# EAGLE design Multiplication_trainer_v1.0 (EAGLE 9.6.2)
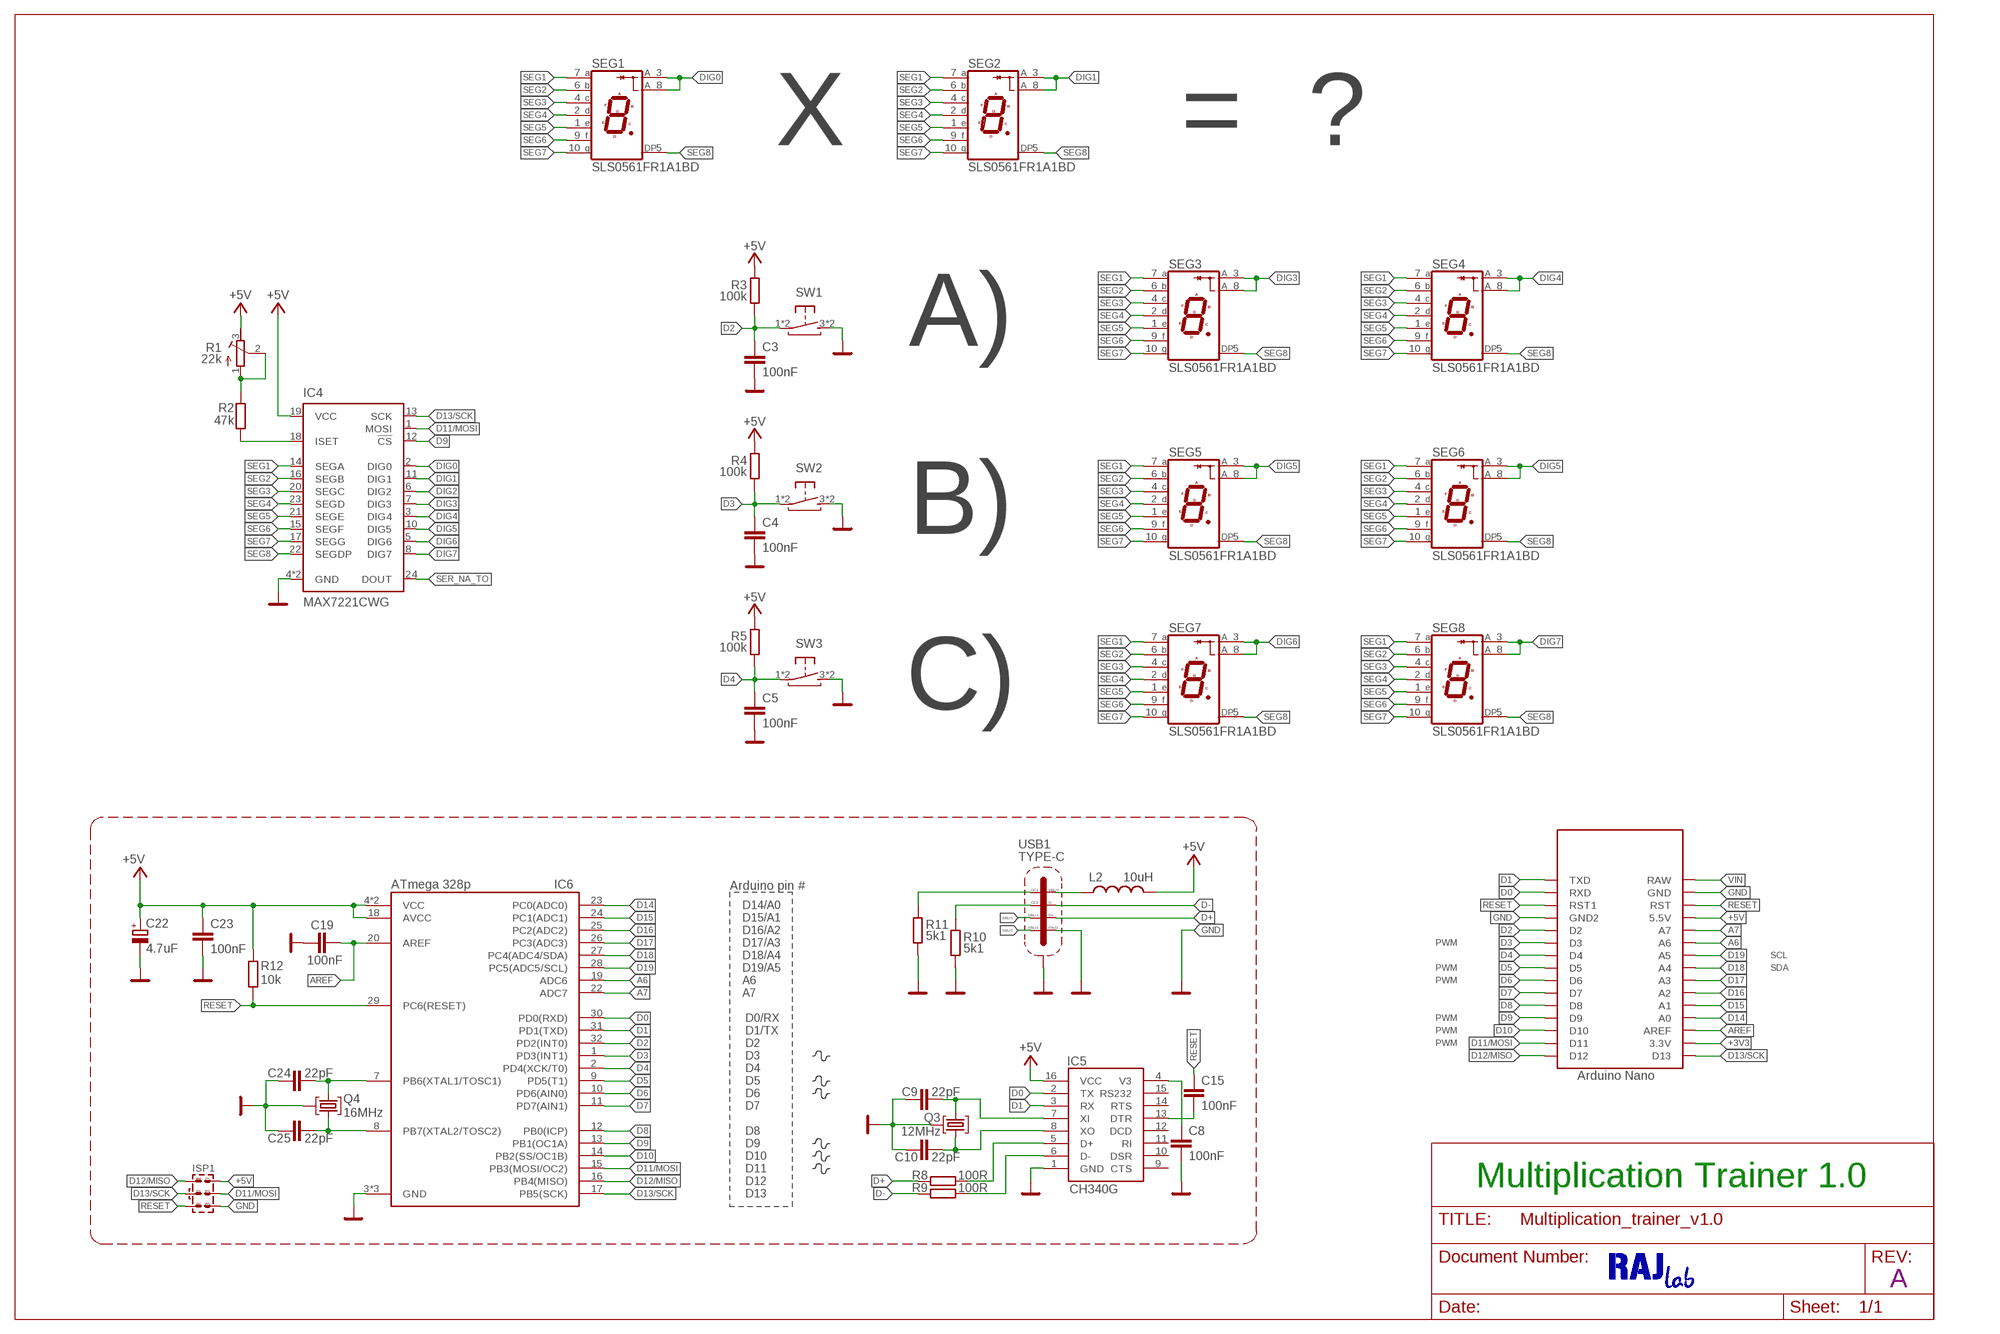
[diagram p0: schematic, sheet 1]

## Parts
C3  100nF  C-EUC0805  [C0805]
C4  100nF  C-EUC0805  [C0805]
C5  100nF  C-EUC0805  [C0805]
C8  100nF  C-EUC0603  [C0603]
C9  22pF  C-EUC0603  [C0603]
C10  22pF  C-EUC0603  [C0603]
C15  100nF  C-EUC0603  [C0603]
C19  100nF  C-EUC0603  [C0603]
C22  4.7uF  CPOL-EUSMCA  [SMC_A]
C23  100nF  C-EUC0603  [C0603]
C24  22pF  C-EUC0603  [C0603]
C25  22pF  C-EUC0603  [C0603]
IC4  MAX7221CWG  [SOIC127P1032X265-24N]
IC5  CH340G  CH340GSMD  [SOIC16]
IC6  ATmega 328p  ATMEGA328PQFP32N_ROUND-PADS  [QFP80P900X900X120-32N_ROUND-PADS]
ISP1  AVR-ISP-SPI  [AVR-ISP-SPI]
L2  10uH  L-USL0805  [R0805]
Q3  12MHz  KRYSTAL  [ILCX13-FF5F18-16.0000]
Q4  16MHz  KRYSTAL  [ILCX13-FF5F18-16.0000]
R1  22k  R-TRIMM3305  [RTRIM3305]
R2  47k  R-EU_R0805  [R0805]
R3  100k  R-EU_R0805  [R0805]
R4  100k  R-EU_R0805  [R0805]
R5  100k  R-EU_R0805  [R0805]
R8  100R  R-EU_R0603  [R0603]
R9  100R  R-EU_R0603  [R0603]
R10  5k1  R-EU_R0603  [R0603]
R11  5k1  R-EU_R0603  [R0603]
R12  10k  R-EU_R0603  [R0603]
SEG1  SLS0561FR1A1BD  [SLS0561FR1A1BD]
SEG2  SLS0561FR1A1BD  [SLS0561FR1A1BD]
SEG3  SLS0561FR1A1BD  [SLS0561FR1A1BD]
SEG4  SLS0561FR1A1BD  [SLS0561FR1A1BD]
SEG5  SLS0561FR1A1BD  [SLS0561FR1A1BD]
SEG6  SLS0561FR1A1BD  [SLS0561FR1A1BD]
SEG7  SLS0561FR1A1BD  [SLS0561FR1A1BD]
SEG8  SLS0561FR1A1BD  [SLS0561FR1A1BD]
SW1  TACT-SW_BTNSMTJLC_6X6X4.5  [TACTSW_6X6X4.5_SMT]
SW2  TACT-SW_BTNSMTJLC_6X6X4.5  [TACTSW_6X6X4.5_SMT]
SW3  TACT-SW_BTNSMTJLC_6X6X4.5  [TACTSW_6X6X4.5_SMT]
U$2  NANOTHT-NOUSB  [NANO-NOUSB]
USB1  TYPE-C  TYPE-C-31-M-12TYPE-C-31_L8.94_W7.3  [TYPE-C-31_L8.94_W7.3]

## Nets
+3V3: U$2.3.3V
+5V: C22.+ C23.1 IC4.19(VCC) IC5.16(VCC) IC6.4(VCC) IC6.6(VCC) IC6.18(AVCC) ISP1.2 L2.2 R1.3(E) R3.1 R4.1 R5.1 R12.1 U$2.5V(5.5V)
A6: IC6.19(ADC6) U$2.A6
A7: IC6.22(ADC7) U$2.A7
AREF: C19.1 IC6.20(AREF) U$2.AREF
D0: IC5.2(TX) IC6.30(PD0(RXD)) U$2.RX1(RXD)
D1: IC5.3(RX) IC6.31(PD1(TXD)) U$2.TX0(TXD)
D2: C3.1 IC6.32(PD2(INT0)) R3.2 SW1.1(P) SW1.2(P) U$2.D2
D3: C4.1 IC6.1(PD3(INT1)) R4.2 SW2.1(P) SW2.2(P) U$2.D3
D4: C5.1 IC6.2(PD4(XCK/T0)) R5.2 SW3.1(P) SW3.2(P) U$2.D4
D5: IC6.9(PD5(T1)) U$2.D5
D6: IC6.10(PD6(AIN0)) U$2.D6
D7: IC6.11(PD7(AIN1)) U$2.D7
D8: IC6.12(PB0(ICP)) U$2.D8
D9: IC4.12(!CS) IC6.13(PB1(OC1A)) U$2.D9
D10: IC6.14(PB2(SS/OC1B)) U$2.D10
D11/MOSI: IC4.1(MOSI) IC6.15(PB3(MOSI/OC2)) ISP1.4 U$2.D11
D12/MISO: IC6.16(PB4(MISO)) ISP1.1 U$2.D12
D13/SCK: IC4.13(SCK) IC6.17(PB5(SCK)) ISP1.3 U$2.D13
D14: IC6.23(PC0(ADC0)) U$2.A0
D15: IC6.24(PC1(ADC1)) U$2.A1
D16: IC6.25(PC2(ADC2)) U$2.A2
D17: IC6.26(PC3(ADC3)) U$2.A3
D18: IC6.27(PC4(ADC4/SDA)) U$2.A4
D19: IC6.28(PC5(ADC5/SCL)) U$2.A5
D+: R8.1 USB1.A6(D+) USB1.B6(D+)
D-: R9.1 USB1.A7(D-) USB1.B7(D-)
DIG0: IC4.2(DIG0) SEG1.3(CA1) SEG1.8(CA2)
DIG1: IC4.11(DIG1) SEG2.3(CA1) SEG2.8(CA2)
DIG2: IC4.6(DIG2)
DIG3: IC4.7(DIG3) SEG3.3(CA1) SEG3.8(CA2)
DIG4: IC4.3(DIG4) SEG4.3(CA1) SEG4.8(CA2)
DIG5: IC4.10(DIG5) SEG5.3(CA1) SEG5.8(CA2) SEG6.3(CA1) SEG6.8(CA2)
DIG6: IC4.5(DIG6) SEG7.3(CA1) SEG7.8(CA2)
DIG7: IC4.8(DIG7) SEG8.3(CA1) SEG8.8(CA2)
GND: C3.2 C4.2 C5.2 C8.2 C9.2 C10.2 C19.2 C22.- C23.2 C24.2 C25.2 IC4.4(GND) IC4.9(GND) IC5.1(GND) IC6.3(GND) IC6.5(GND) IC6.21(GND) ISP1.6 Q3.P$2(GND) Q3.P$4(GND) Q4.P$2(GND) Q4.P$4(GND) R10.1 R11.1 SW1.3(S) SW1.4(S) SW2.3(S) SW2.4(S) SW3.3(S) SW3.4(S) U$2.GND U$2.GND1(GND2) USB1.A1/B12(GND) USB1.B1/A12(GND) USB1.SHIELD1(SHIELD) USB1.SHIELD2(SHIELD) USB1.SHIELD3(SHIELD) USB1.SHIELD4(SHIELD) USB1.SHIELD5(SHIELD) USB1.SHIELD6(SHIELD) USB1.SHIELD7(SHIELD) USB1.SHIELD8(SHIELD)
N$1: C8.1 IC5.4(V3)
N$2: C9.1 IC5.7(XI) Q3.P$1
N$3: C10.1 IC5.8(XO) Q3.P$3
N$4: C15.2 IC5.13(DTR)
N$5: IC5.5(D+) R8.2
N$6: IC4.18(ISET) R2.1
N$7: R1.1(A) R1.2(S) R2.2
N$8: IC5.6(D-) R9.2
N$9: L2.1 USB1.A4/B9(VBUS) USB1.B4/A9(VBUS)
N$10: R10.2 USB1.B5(CC2)
N$11: R11.2 USB1.A5(CC1)
N$12: C24.1 IC6.7(PB6(XTAL1/TOSC1)) Q4.P$1
N$13: C25.1 IC6.8(PB7(XTAL2/TOSC2)) Q4.P$3
RESET: C15.1 IC6.29(PC6(RESET)) ISP1.5 R12.2 U$2.RST U$2.RST1
SBU1: USB1.A8(SBU1)
SBU2: USB1.B8(SBU2)
SEG1: IC4.14(SEGA) SEG1.7(A) SEG2.7(A) SEG3.7(A) SEG4.7(A) SEG5.7(A) SEG6.7(A) SEG7.7(A) SEG8.7(A)
SEG2: IC4.16(SEGB) SEG1.6(B) SEG2.6(B) SEG3.6(B) SEG4.6(B) SEG5.6(B) SEG6.6(B) SEG7.6(B) SEG8.6(B)
SEG3: IC4.20(SEGC) SEG1.4(C) SEG2.4(C) SEG3.4(C) SEG4.4(C) SEG5.4(C) SEG6.4(C) SEG7.4(C) SEG8.4(C)
SEG4: IC4.23(SEGD) SEG1.2(D) SEG2.2(D) SEG3.2(D) SEG4.2(D) SEG5.2(D) SEG6.2(D) SEG7.2(D) SEG8.2(D)
SEG5: IC4.21(SEGE) SEG1.1(E) SEG2.1(E) SEG3.1(E) SEG4.1(E) SEG5.1(E) SEG6.1(E) SEG7.1(E) SEG8.1(E)
SEG6: IC4.15(SEGF) SEG1.9(F) SEG2.9(F) SEG3.9(F) SEG4.9(F) SEG5.9(F) SEG6.9(F) SEG7.9(F) SEG8.9(F)
SEG7: IC4.17(SEGG) SEG1.10(G) SEG2.10(G) SEG3.10(G) SEG4.10(G) SEG5.10(G) SEG6.10(G) SEG7.10(G) SEG8.10(G)
SEG8: IC4.22(SEGDP) SEG1.5(DP) SEG2.5(DP) SEG3.5(DP) SEG4.5(DP) SEG5.5(DP) SEG6.5(DP) SEG7.5(DP) SEG8.5(DP)
SER_NA_TO: IC4.24(DOUT)
VIN: U$2.RAW
Unconnected: IC5.9(CTS) IC5.10(DSR) IC5.11(RI) IC5.12(DCD) IC5.14(RTS) IC5.15(RS232)

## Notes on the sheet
- X | = | ?
- A)
- B)
- C)
- Arduino pin #
- D14/A0
- D15/A1
- D16/A2
- D17/A3 | PWM
- D18/A4 | SCL
- D19/A5 | PWM | SDA
- A6 | PWM
- A7
- D0/RX | PWM
- D1/TX | PWM
- D2 | PWM
- D3
- D4
- D5
- D6
- D7
- D8
- D9
- D10
- D11
- D12
- Multiplication Trainer 1.0
- D13
- A

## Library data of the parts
C3-C5 = rcl:C-EU: CAPACITOR, European symbol
C8 C15 C19 C23 = rcl:C-EU: CAPACITOR, European symbol; LCSC_PART: C49678; SPICEPREFIX: C
C9 C10 C24 C25 = rcl:C-EU: CAPACITOR, European symbol; LCSC_PART: C1804; SPICEPREFIX: C
C22 = rcl:CPOL-EU: POLARIZED CAPACITOR, European symbol; LCSC_PART: C111040; ROT: 180; SPICEPREFIX: C
IC4 = MAX7221:MAX7221CWG: 7 SEGMENT 8 DIGIT DRIVER 24SOIC Datasheet; MOUSER_NO: 710-157119S12701
IC5 = ch340g:CH340G; LCSC_PART: C14267
IC6 = ATMEGA328P-ANR:ATMEGA328P: 8-bit Microcontrollers - MCU AVR 32K FLSH 2K SRAM 1KB EE-20 MHZ 105C Source: Datasheet; LCSC_PART: C14877; ROT: 270
ISP1 = #Ondra2:AVR-ISP-SPI
L2 = rcl:L-US: INDUCTOR, American symbol; LCSC_PART: C281113
Q3 = #Marek:KRYSTAL: Monolithic Crystal Filters Source: www.vanlong.com; LCSC_PART: C9002
Q4 = #Marek:KRYSTAL: Monolithic Crystal Filters Source: www.vanlong.com; LCSC_PART: C13738
R1 = rcl:R-TRIMM: Trimm resistor
R2 R8 R9 R12 = rcl:R-EU_: RESISTOR, European symbol; SPICEPREFIX: R
R3-R5 = resistor:R-EU_: RESISTOR, European symbol
R10 R11 = rcl:R-EU_: RESISTOR, European symbol; LCSC_PART: C27834; SPICEPREFIX: R
SEG1-SEG8 = #my:SLS0561FR1A1BD; LCSC_PART: C226002
SW1-SW3 = #Ondra2:TACT-SW_BTN; LCSC_PART: C127509
U$2 = Arduino-clone:NANO: Arduino Nano
USB1 = #Marek:TYPE-C-31-M-12; LCSC_PART: C165948; ROT: 180

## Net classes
0 default: width 0.127 mm, drill 0.2 mm, clearance 0.127 mm

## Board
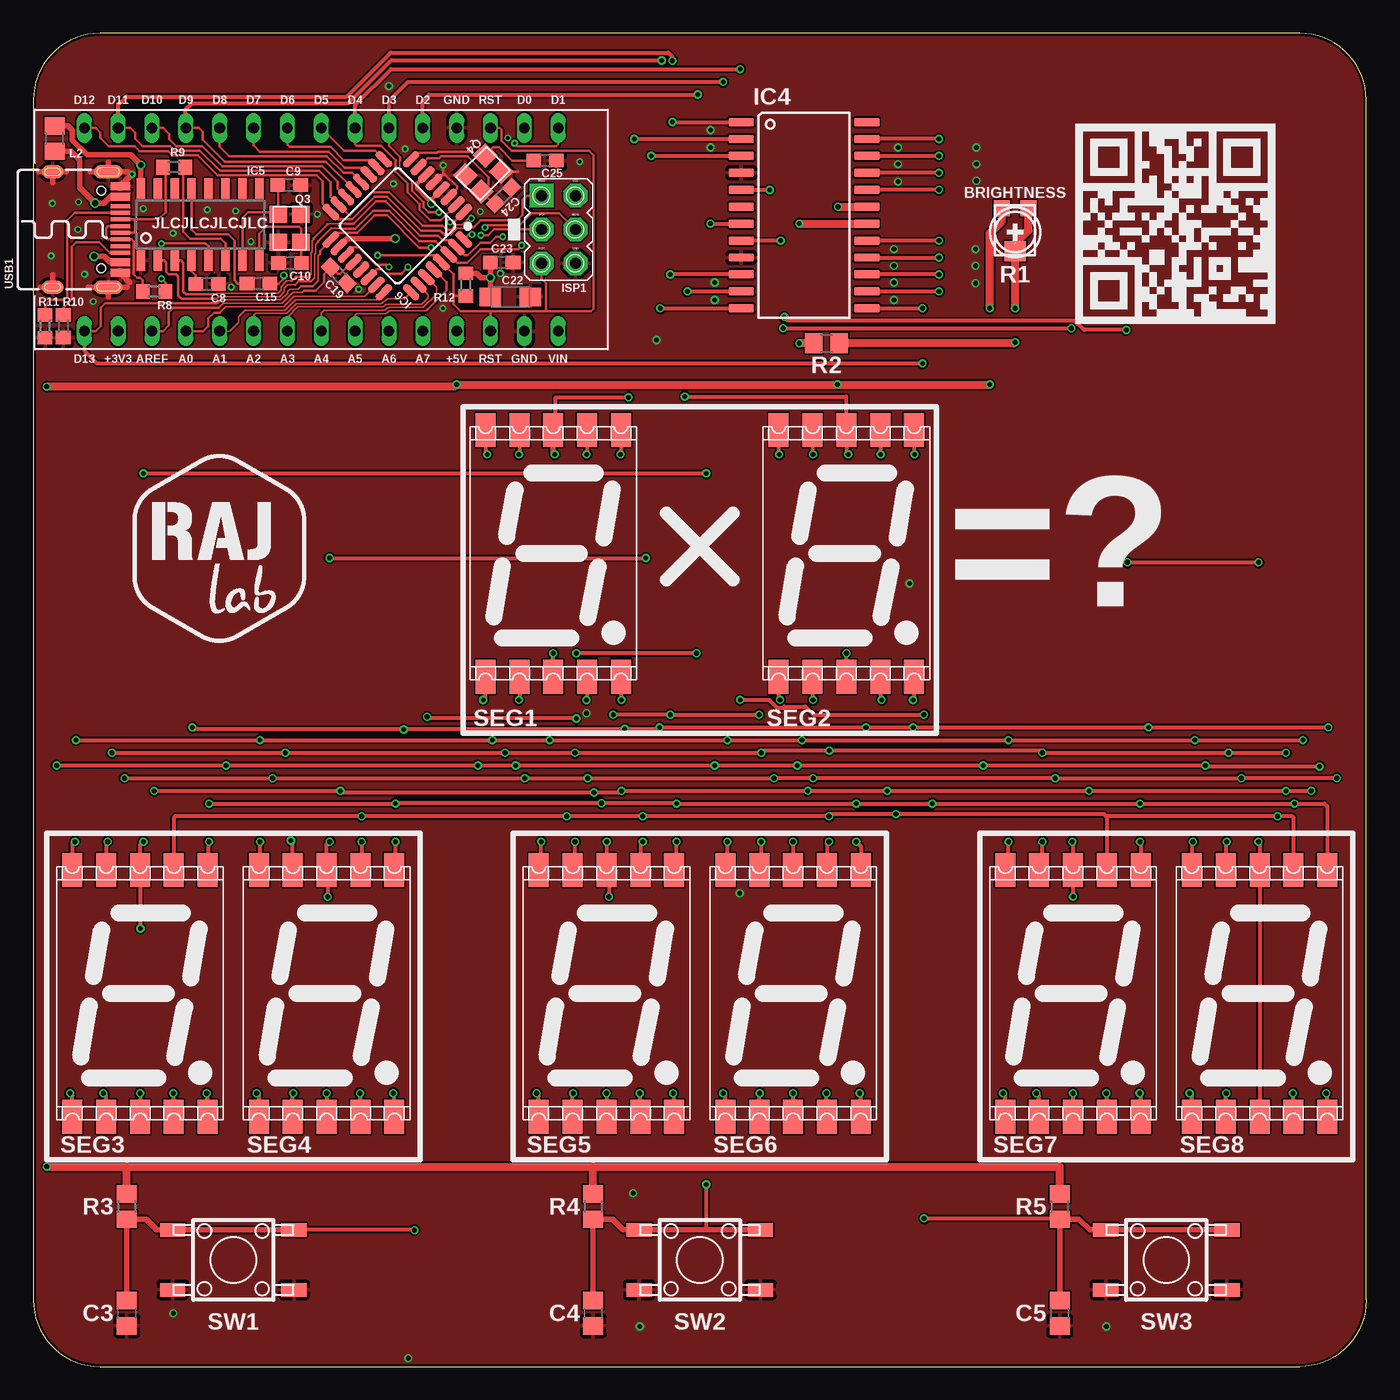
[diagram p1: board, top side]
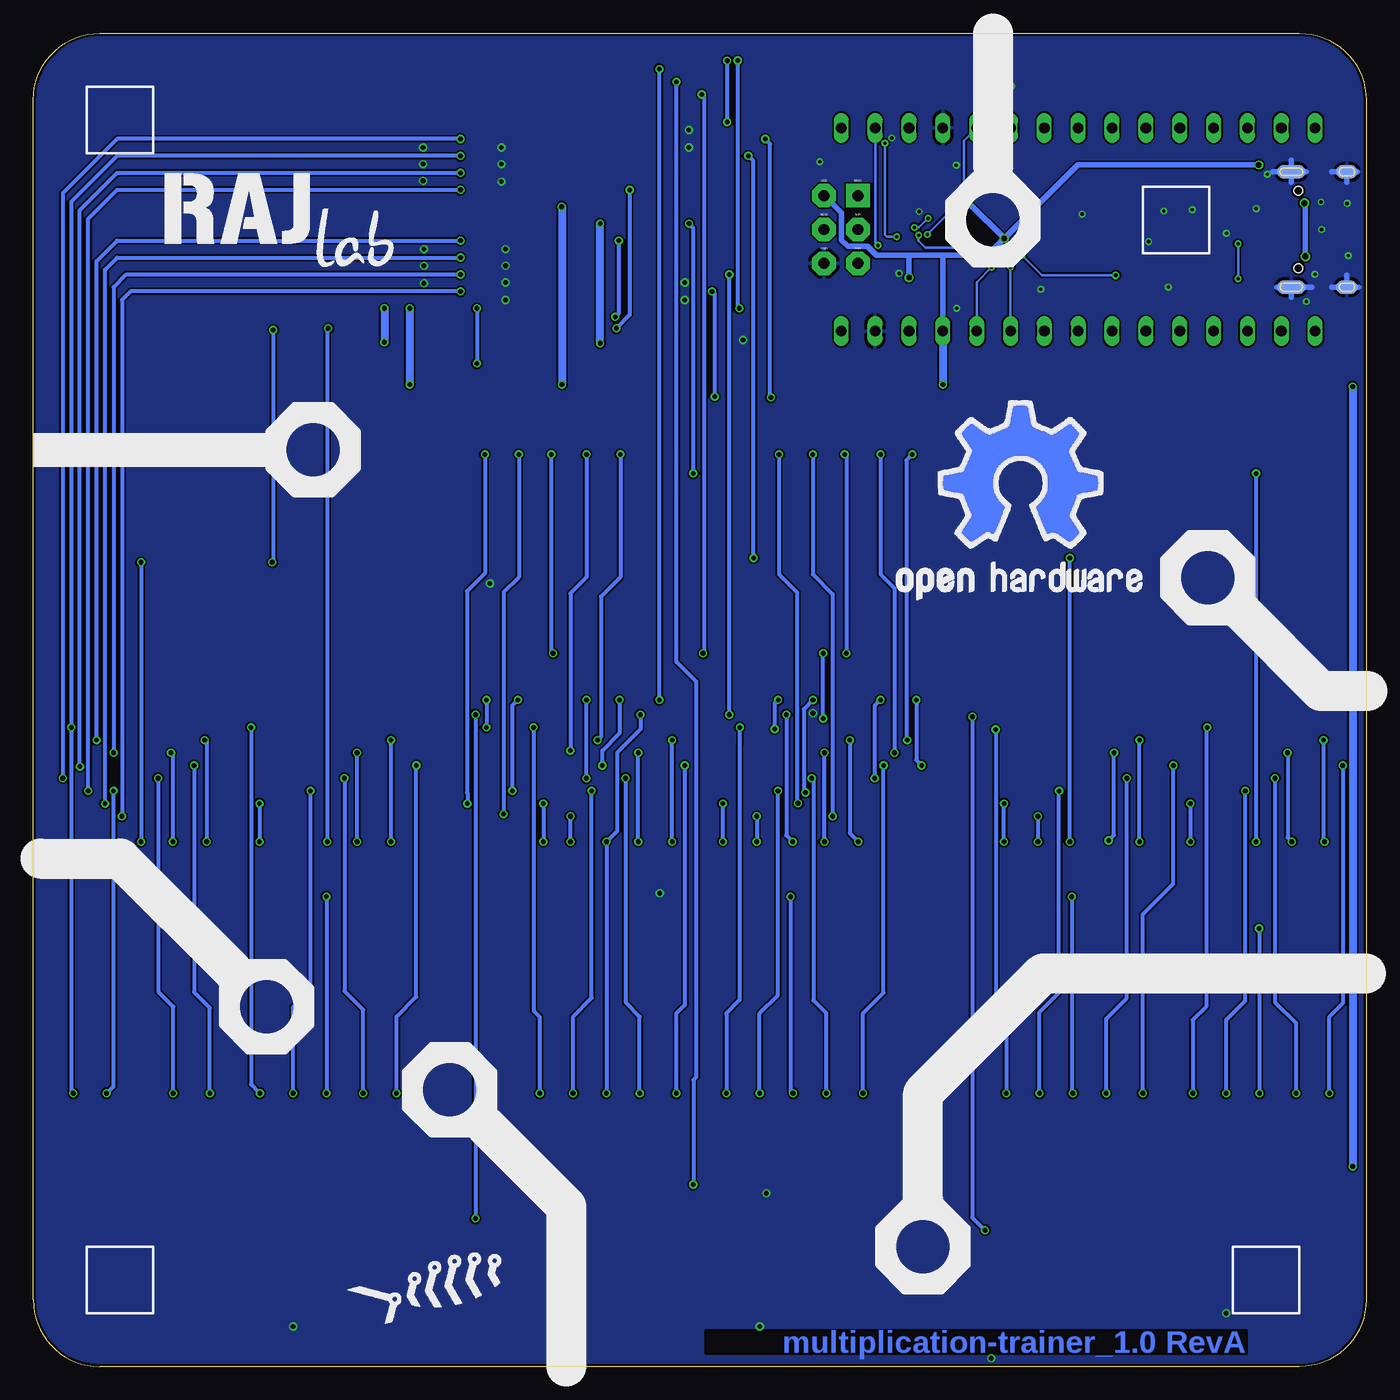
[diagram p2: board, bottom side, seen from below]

Size 100 x 100 mm. Coordinates in mm from the lower left corner, seen from the top.
Outline: 100,5 100,95 arc90 95,100 5,100 arc90 0,95 0,5 arc90 5,0 95,0 arc90 100,5
Copper layers (1*16): Top 0.035mm / dielectric 1.6mm / Bottom 0.035mm
Design rules "jlcpcb-2layers_od-Ondry3-assembly-tight": minimum track width 5mil, minimum drill 0.2mm, track to track 5mil, track to pad 5mil, pad to pad 5mil, via to via 5mil, smd to smd 5mil, copper to edge 0.2mm, drill to drill 6mil, minimum pad ring 0.13mm, minimum via ring 0.13mm, stop-mask expansion 4mil, vias tented up to drill 0.6mm, thermal gap 10mil

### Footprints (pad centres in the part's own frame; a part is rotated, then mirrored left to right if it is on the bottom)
C0805 = smd 1.3 x 1.5: 1 -0.95,0; 2 0.95,0
C0603 = smd 1.1 x 1: 1 -0.85,0; 2 0.85,0
SMC_A = smd 1.6 x 1.4: + -1.5,0; - 1.5,0
SOIC127P1032X265-24N = smd 1.925 x 0.65: 1 -4.712,6.985; 2 -4.712,5.715; 3 -4.712,4.445; 4 -4.712,3.175; 5 -4.712,1.905; 6 -4.712,0.635; 7 -4.712,-0.635; 8 -4.712,-1.905; 9 -4.712,-3.175; 10 -4.712,-4.445; 11 -4.712,-5.715; 12 -4.712,-6.985; 13 4.712,-6.985; 14 4.712,-5.715; 15 4.712,-4.445; 16 4.712,-3.175; 17 4.712,-1.905; 18 4.712,-0.635; 19 4.712,0.635; 20 4.712,1.905; 21 4.712,3.175; 22 4.712,4.445; 23 4.712,5.715; 24 4.712,6.985
SOIC16 = smd 0.635 x 1.524: 1 -4.445,-2.695; 2 -3.175,-2.695; 3 -1.905,-2.695; 4 -0.635,-2.695; 5 0.635,-2.695; 6 1.905,-2.695; 7 3.175,-2.695; 8 4.445,-2.695; 9 4.445,2.695; 10 3.175,2.695; 11 1.905,2.695; 12 0.635,2.695; 13 -0.635,2.695; 14 -1.905,2.695; 15 -3.175,2.695; 16 -4.445,2.695
QFP80P900X900X120-32N_ROUND-PADS = smd 1.499 x 0.584: 1 -4.25,2.8; 2 -4.25,2; 3 -4.25,1.2; 4 -4.25,0.4; 5 -4.25,-0.4; 6 -4.25,-1.2; 7 -4.25,-2; 8 -4.25,-2.8; 17 4.25,-2.8; 18 4.25,-2; 19 4.25,-1.2; 20 4.25,-0.4; 21 4.25,0.4; 22 4.25,1.2; 23 4.25,2; 24 4.25,2.8 | smd 0.584 x 1.499: 9 -2.8,-4.25; 10 -2,-4.25; 11 -1.2,-4.25; 12 -0.4,-4.25; 13 0.4,-4.25; 14 1.2,-4.25; 15 2,-4.25; 16 2.8,-4.25; 25 2.8,4.25; 26 2,4.25; 27 1.2,4.25; 28 0.4,4.25; 29 -0.4,4.25; 30 -1.2,4.25; 31 -2,4.25; 32 -2.8,4.25
AVR-ISP-SPI = drill 0.813 pad 1.778 square: 1 -1.27,2.54 | drill 0.813 pad 1.778 octagon: 2 1.27,2.54; 3 -1.27,0; 4 1.27,0; 5 -1.27,-2.54; 6 1.27,-2.54
R0805 = smd 1.3 x 1.5: 1 -0.95,0; 2 0.95,0
ILCX13-FF5F18-16.0000 = smd 1.3 x 1.3: P$1 -1.05,-0.85; P$2 1.05,-0.85; P$3 1.05,0.85; P$4 -1.05,0.85
RTRIM3305 = smd 1.2 x 1.2: 1 -1,-1.8; 3 1,-1.8 | smd 1.6 x 1.5: 2 0,1.45
R0603 = smd 1 x 1.1: 1 -0.85,0; 2 0.85,0
SLS0561FR1A1BD = smd 1.5 x 2.54: 1 -5.08,-9.25; 2 -2.54,-9.25; 3 0,-9.25; 4 2.54,-9.25; 5 5.08,-9.25; 6 5.08,9.25; 7 2.54,9.25; 8 0,9.25; 9 -2.54,9.25; 10 -5.08,9.25
TACTSW_6X6X4.5_SMT = smd 1.9 x 1: 1 -4.55,2.25; 2 4.55,2.25; 3 -4.55,-2.25; 4 4.55,-2.25
NANO-NOUSB = drill 0.8 long: 3.3V -7.62,15.24; 5V -7.62,-10.16; A0 -7.62,10.16; A1 -7.62,7.62; A2 -7.62,5.08; A3 -7.62,2.54; A4 -7.62,0; A5 -7.62,-2.54; A6 -7.62,-5.08; A7 -7.62,-7.62; AREF -7.62,12.7; D2 7.62,-7.62; D3 7.62,-5.08; D4 7.62,-2.54; D5 7.62,0; D6 7.62,2.54; D7 7.62,5.08; D8 7.62,7.62; D9 7.62,10.16; D10 7.62,12.7; D11 7.62,15.24; D12 7.62,17.78; D13 -7.62,17.78; GND -7.62,-15.24; GND1 7.62,-10.16; RAW -7.62,-17.78; RST -7.62,-12.7; RST1 7.62,-12.7; RX1 7.62,-15.24; TX0 7.62,-17.78
TYPE-C-31_L8.94_W7.3 = smd 0.6 x 1.45: A1/B12 -3.25,3.885; A4/B9 -2.45,3.885; B1/A12 3.25,3.885; B4/A9 2.45,3.885 | smd 0.3 x 1.45: A5 -1.25,3.885; A6 -0.25,3.885; A7 0.25,3.885; A8 1.25,3.885; B5 1.75,3.885; B6 0.75,3.885; B7 -0.75,3.885; B8 -1.75,3.885 | smd 1 x 2.1: SHIELD1 -4.32,2.97; SHIELD2 4.32,2.97 | smd 1 x 1.6: SHIELD3 -4.32,-1.21; SHIELD4 4.32,-1.21 | smd 1 x 2.1 bottom: SHIELD5 -4.316,2.97; SHIELD8 4.316,2.97 | smd 1 x 1.6 bottom: SHIELD6 -4.316,-1.21; SHIELD7 4.316,-1.21 | hole 0.65: -2.89,2.44; 2.89,2.44

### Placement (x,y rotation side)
C3  7,4 270 top
C4  42,4 270 top
C5  77,4 270 top
C8  13.04,81.2 0 top
C9  19.19,88.62 0 top
C10  19.25,82.78 180 top
C15  16.89,81.24 180 top
C19  22.91,81.85 315 top
C22  35.79,80.23 0 top
C23  35.14,82.82 0 top
C24  35.26,87.83 45 top
C25  38.39,90.46 0 top
IC4  57.82,86.36 0 top
IC5  12.51,85.66 0 top
IC6  27.31,85.56 225 top
ISP1  39.4,85.29 0 top
L2  1.59,92.11 90 top
Q3  19.22,85.38 270 top
Q4  33.75,89.49 45 top
R1  73.66,85.09 180 top
R2  59.5,76.75 0 top
R3  7,12 270 top
R4  42,12 270 top
R5  77,12 270 top
R8  9.06,80.62 0 top
R9  10.56,89.96 0 top
R10  2.24,78.02 90 top
R11  0.87,78.02 90 top
R12  32.44,81.15 270 top
SEG1  39,61 0 top
SEG2  61,61 0 top
SEG3  8,28 0 top
SEG4  22,28 0 top
SEG5  43,28 0 top
SEG6  57,28 0 top
SEG7  78,28 0 top
SEG8  92,28 0 top
SW1  15,8 0 top
SW2  50,8 0 top
SW3  85,8 0 top
U$1  [DESIGN-PAD]  79,68.75 0 bottom
U$2  21.6,85.29 90 top
U$3  [OPEN-HARDWARE_15MM_TEXT]  26,65 0 bottom
U$4  [DESIGN-PAD]  82.5,27 0 bottom
U$5  [DESIGN-PAD]  68.75,20.75 0 bottom
U$6  [DESIGN-PAD]  33.25,9 0 bottom
U$8  [RYBICKA_12MM]  69,6 0 bottom
U$10  [DESIGN-PAD]  28,86 180 bottom
U$19  [RAJLAB-HEX_15MM_N]  14,61 0 top
U$21  [RAJLAB-TEXT_7MM]  79,85 0 bottom
U$22  [DESIGN-PAD]  11.88,59.18 180 bottom
USB1  2.64,85.29 270 top

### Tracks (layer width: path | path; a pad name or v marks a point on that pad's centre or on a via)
+5V  (via drill 0.35, 0.35 pad 0.55, 0.4)
  Top 0.305: IC6.4 29.84,87.52 | 29.85,87.52 29.84,87.52 | 29.84,87.52 29.62,87.52 28.78,88.36 28.78,88.73 IC6.6
  Top 0.406: L2.2 2.59,93.06 2.93,92.72 2.93,91.98 4.02,90.88 7.3,90.88 v8.06,90.13 IC5.16 | IC6.18 23.52,84.6 27.13,84.6 v27.15,84.61 | v29.85,87.24 29.85,87.52 | C22.+ v34.29,81.67 | v34.29,81.67 v34.29,81.68 | C23.1 v34.29,81.67 | v34.29,81.67 | R12.1 33.25,82 33.58,81.67 v34.29,81.67
  Top 0.61: R3.1 7,15 | R4.1 42,15 | R5.1 77,15 42,15 | v1,15 7,15 | 7,15 42,15 | v1,73.5 31.59,73.5 v31.75,73.66 v60.33,73.66 v71.75,73.66 | v60.36,87 IC4.19 | v71.75,79.38 71.75,85.01 72.66,85.91 R1.3
  Bottom 0.406: v27.15,84.61 29.77,87.24 v29.85,87.24 | v27.15,84.61 28.42,83.34 31.75,83.34 | v34.29,81.68 34.29,83.26 34.21,83.34 | 31.75,83.34 34.21,83.34 | 34.21,83.34 36.74,83.34 37.42,84.02 38.89,84.02 39.37,84.5 39.37,86.53 ISP1.2 | v27.15,84.61 21.63,90.13 v8.06,90.13 | U$2.5V 31.76,83.33 31.75,83.34
  Bottom 0.61: U$2.5V v31.76,73.67 v31.75,73.66 | v60.36,87 60.33,86.96 v60.33,73.66 | v1,73.5 v1,15 | v71.75,79.38 v71.75,73.66
A6  (via drill 0.25)
  Top 0.203: IC6.19 24.02,83.96 24.39,83.96 25.72,82.63 26.51,82.63 v26.67,82.47
  Bottom 0.203: U$2.A6 v26.68,82.47 v26.67,82.47
A7  (via drill 0.25)
  Top 0.203: IC6.22 25.75,82.3 26.13,82.3 26.44,81.98 27.61,81.98 v28.09,82.46 v28.1,82.46
  Bottom 0.203: U$2.A7 29.22,81.34 v28.1,82.46
AREF
  Top 0.127: 13.89,79.42 14.22,79.75 18.67,79.75 19.49,80.57 20.16,80.57 20.3,80.71
  Top 0.203: U$2.AREF 9.72,77.67 10.16,78.1 10.16,79.09 10.49,79.42 13.89,79.42 | 20.3,80.71 21.16,80.71 21.8,81.34 21.8,81.94 C19.1 22.81,81.95 23.02,81.95 23.91,82.84 IC6.20
D0  (via drill 0.25)
  Top 0.127: 22.35,85.4 23.2,85.4 23.24,85.36 | 13.65,80.08 13.73,80.08 13.91,80.26 18.46,80.26 18.82,80.62 18.82,80.88 19.08,81.14 19.63,81.14 | 20.82,81.39 21.09,81.66 21.09,83.42 21.17,83.5 21.17,84.17 21.37,84.37
  Top 0.203: 13.65,80.08 11.11,80.08 10.87,80.32 10.87,81.76 10.72,81.92 10.16,81.92 9.97,82.11 9.97,82.8 9.81,82.96 IC5.2 | v36.63,84.1 36.35,83.81 33.55,83.81 32.53,82.79 31.79,82.79 IC6.30 30.16,84.42 28.93,84.42 26.67,86.68 25.47,86.68 24.15,85.36 23.24,85.36 | 22.35,85.4 21.37,84.41 21.37,84.37 | 19.63,81.14 19.89,81.39 20.82,81.39
  Bottom 0.203: v36.63,84.1 36.83,84.3 36.83,92.9 U$2.RX1
D1  (via drill 0.25)
  Top 0.127: 22.03,85.68 22.07,85.72 23.36,85.72 23.37,85.72 | 13.57,80.41 13.65,80.41 13.75,80.51 18.36,80.51 18.57,80.73 18.57,80.98 19.02,81.43 19.38,81.43 | 20.62,81.74 20.84,81.96 20.84,83.53 20.91,83.61 20.91,84.43 21.03,84.54
  Top 0.203: 21.03,84.54 21.03,84.62 22.09,85.68 22.03,85.68 | 23.37,85.72 24.03,85.72 25.72,87.41 26.41,87.41 29.01,84.81 30.38,84.81 30.72,84.47 31.24,84.47 IC6.31 32.37,83.34 32.57,83.34 33.53,84.3 34.27,84.3 34.71,84.74 v35.23,84.74 | v36.1,91.76 36.34,91.52 39.22,91.52 39.38,91.68 U$2.TX0 | 20.62,81.74 19.69,81.74 19.38,81.43 | IC5.3 11.08,82.96 11.24,82.8 11.24,80.62 11.44,80.41 13.57,80.41
  Bottom 0.203: v35.23,84.74 35.95,84.74 36.1,84.89 v36.1,91.76
D2  (via drill 0.25, 0.35)
  Top 0.203: IC6.32 32.66,84.9 32.91,84.9 v32.92,84.91
  Top 0.305: U$2.D2 29.22,94.94 29.69,95.41 v49.85,95.41 | v28.59,10.23 28.57,10.25 SW1.2 | v49.75,53.5 v40.73,53.5 | v29.54,48.74 29.67,48.61 v40.73,48.61
  Top 0.406: SW1.2 SW1.1 9.25,10.25 8.45,11.05 R3.2 C3.1
  Bottom 0.203: v32.92,84.91 32.78,85.04 32.78,85.1 30.17,87.7 30.17,91.95 U$2.D2
  Bottom 0.305: v29.54,48.74 29.54,11.18 v28.59,10.23 | v49.85,95.41 49.69,95.25 49.69,53.56 v49.75,53.5 | v40.73,48.61 v40.73,53.5
D3  (via drill 0.25, 0.35)
  Top 0.127: 27.55,89.7 27.46,89.79 27.46,90.45 27.51,90.5
  Top 0.203: IC6.1 31.64,85.93 31.34,85.93 v31.26,85.85 | v30.41,86.58 29.66,86.58 29.29,86.94 29.29,87.31 28.4,88.21 28.4,88.86 27.55,89.7 | 27.51,90.5 27.51,90.72 26.68,91.56 U$2.D3
  Top 0.305: U$2.D3 26.68,94.94 28.1,96.36 v51.75,96.36 | v50.48,13.65 50.48,10.25
  Top 0.406: C4.1 R4.2 43.45,11.05 44.25,10.25 SW2.1 50.48,10.25 SW2.2
  Bottom 0.203: v31.26,85.85 30.54,86.58 v30.41,86.58
  Bottom 0.305: v50.48,13.65 50.48,21.51 50.25,21.73 50.25,51.37 51.75,52.86 v51.75,96.36
D4  (via drill 0.35)
  Top 0.203: U$2.D4 24.14,91.67 24.25,91.56 26.07,91.56 27.16,90.48 27.16,89.63 28.07,88.72 28.07,88.07 28.96,87.18 28.96,86.81 28.97,86.8 28.97,86.76 29.77,85.96 30.54,85.96 IC6.2
  Top 0.305: U$2.D4 24.14,94.62 26.83,97.31 v53.02,97.31 | v66.82,11.11 76.94,11.11 R5.2 | v66.82,48.9 58.53,48.9 57.92,49.51 56.34,49.51 56.26,49.42 55.78,49.42 55.19,50.01 v53.02,50.01
  Top 0.406: SW3.2 SW3.1 79.25,10.25 78.45,11.05 R5.2 C5.1
  Bottom 0.305: v66.82,48.9 v66.82,11.11 | v53.02,50.01 v53.02,97.31
D5
  Top 0.203: IC6.9 25.64,91.2 23.3,91.2 U$2.D5
D6
  Top 0.203: IC6.10 25.21,90.5 23.29,90.5 22.31,91.48 19.22,91.48 19.06,91.64 U$2.D6
D7
  Top 0.203: IC6.11 25.11,89.42 24.6,89.93 23.34,89.93 22.16,91.12 16.99,91.12 16.52,91.59 U$2.D7
D8
  Top 0.203: U$2.D8 13.98,91.5 14.68,90.79 22.02,90.79 23.28,89.53 23.92,89.53 IC6.12
D9  (via drill 0.35)
  Top 0.203: U$2.D9 12.42,92.91 12.7,92.62 12.7,92.02 14.33,90.38 21.93,90.38 IC6.13
  Top 0.305: U$2.D9 11.44,94.31 11.91,94.77 23.63,94.77 26.85,97.99 47.12,97.99 v47.15,97.96 | v47.02,79.38 IC4.12
  Bottom 0.305: v47.15,97.96 47.15,79.5 v47.02,79.38
D10
  Top 0.203: IC6.14 22.84,88.34 22.84,88.86 21.67,90.04 14.17,90.04 12.67,91.54 10.71,91.54 10.2,92.06 10.2,92.43 9.72,92.91 U$2.D10
  Top 0.305: U$2.D10
D11/MOSI  (via drill 0.25, 0.35)  (1 unrouted)
  Top 0.127: 32.31,85.77 32.18,85.64 31.68,85.64 31.32,85.28 31.29,85.28
  Top 0.203: U$2.D11 7.25,92.91 7.63,92.53 7.63,92.08 8.18,91.53 10.26,91.53 10.58,91.21 12.48,91.21 14,89.69 21.45,89.69 22.3,88.84 22.3,87.75 IC6.15 23.66,86.39 23.76,86.39 25.43,88.06 26.68,88.06 29.18,85.57 30.72,85.57 31.01,85.28 31.29,85.28 | v32.86,86.12 32.66,86.12 32.31,85.77 | v33.89,85.44 34.07,85.62 36.48,85.62 37.39,86.52 39.44,86.52 ISP1.4
  Top 0.305: U$2.D11 6.36,94.62 6.99,95.25 23.5,95.25 26.8,98.55 47.64,98.55 47.94,98.25 v47.94,97.95 | v47.94,93.34 IC4.1
  Bottom 0.203: v32.86,86.12 33.55,85.44 v33.89,85.44
  Bottom 0.305: v47.94,97.95 v47.94,93.34
D12/MISO
  Top 0.127: 31.35,84.93 31.8,85.38 32.38,85.38
  Top 0.203: U$2.D12 4.67,92.91 5.02,92.56 5.02,92.16 5.64,91.53 7.6,91.53 7.97,91.16 10.12,91.16 10.42,90.86 12.32,90.86 13.82,89.35 21.24,89.35 21.69,88.9 21.69,87.23 IC6.16 22.87,86.05 23.9,86.05 25.58,87.73 26.55,87.73 29.08,85.2 30.53,85.2 30.8,84.93 31.35,84.93 | ISP1.1 37.03,87.83 36.71,87.51 36.71,86.4 36.28,85.97 33.53,85.97 33.03,85.46 32.46,85.46 32.38,85.38
D13/SCK  (via drill 0.25, 0.35)
  Top 0.127: 13.73,79.75 13.81,79.75 14.06,80 18.57,80 19.08,80.52 19.08,80.64 19.26,80.82 19.87,80.82 20.08,81.04 | 20.95,81.04 21.35,81.44 21.35,83.32 21.5,83.47
  Top 0.203: U$2.D13 4.67,77.67 5.05,78.05 5.05,79.43 5.37,79.75 13.73,79.75 | 21.5,83.47 21.5,83.71 IC6.17 22.82,85.03 24.29,85.03 25.61,86.35 26.53,86.35 28.95,83.93 v29.84,83.93 | v33.58,84.85 34.13,84.85 34.57,85.29 ISP1.3 | 20.08,81.04 20.95,81.04
  Top 0.305: U$2.D13 3.82,76.19 4.76,75.25 v66.71,75.25 | IC4.13 v66.71,79.38
  Bottom 0.203: v29.84,83.93 33.05,83.93 33.58,84.45 v33.58,84.85
  Bottom 0.305: v66.71,79.38 v66.71,75.25
D14
  Top 0.127: 13.97,79.06 14.41,79.5 18.78,79.5 19.57,80.29 24.86,80.29 IC6.23
  Top 0.203: U$2.A0 12.75,77.67 13.11,78.02 13.11,78.61 13.55,79.06 13.97,79.06
D15
  Top 0.127: U$2.A1 14.72,77.67 15.4,78.34 15.4,78.74 15.9,79.24 18.88,79.24 19.66,80.02 25.73,80.02 IC6.24
D16
  Top 0.127: U$2.A2 16.52,78.84 16.67,78.99 18.99,78.99 19.73,79.73 26.02,79.73 arc45 26.24,79.82 26.42,80 arc-45 26.64,80.09 27.85,80.09 IC6.25
D17
  Top 0.127: U$2.A3 19.06,78.7 19.83,79.47 26.12,79.47 arc45 26.35,79.57 26.38,79.6 arc-45 26.61,79.69 29.13,79.69 29.61,80.17 29.61,80.41 28.91,81.11 IC6.26
D18
  Top 0.127: U$2.A4 21.6,78.99 21.83,79.22 26.23,79.22 arc45 26.45,79.31 26.49,79.35 arc-45 26.71,79.44 29.24,79.44 30.24,80.44 30.24,80.94 IC6.27
D19
  Top 0.127: U$2.A5 24.14,78.86 24.25,78.97 26.33,78.97 arc45 26.56,79.06 26.59,79.09 arc-45 26.82,79.18 29.47,79.18 29.58,79.29
  Top 0.203: IC6.28 31,81.31 31,80.71 29.58,79.29
D+
  Top 0.203: USB1.A6 5.59,85.54 5.45,85.4 5.45,84.61 5.53,84.54 USB1.B6 7.38,84.54 7.51,84.4 7.51,81.94 7.78,81.68 8.02,81.68 8.21,81.48 R8.1
D-
  Top 0.203: USB1.A7 7.56,85.04 7.64,85.12 7.64,85.9 7.58,85.96 7.5,86.04 | 7.5,86.04 USB1.B7 | R9.1 9.92,89.75 9.92,86.6 9.36,86.04 7.5,86.04
DIG0  (via drill 0.35)
  Top 0.305: SEG1.3 v39,53.5 | v45.09,92.08 IC4.2 | 39.2,70.44 39.2,72.7 v44.66,72.7
  Top 0.406: v39.12,68.42 39,68.54 SEG1.8 39.2,70.44
  Bottom 0.305: v39.12,68.42 39,68.31 v39,53.5 | v44.66,72.7 44.71,72.75 44.71,91.7 v45.09,92.08
DIG1  (via drill 0.35)
  Top 0.305: v49.08,80.64 IC4.11 | v61.13,68.42 61,68.56 SEG2.8 61,72.75 v48.88,72.75 | SEG2.3 v61,53.5
  Bottom 0.305: v61.13,68.42 61.13,53.63 v61,53.5 | v49.08,80.64 48.88,80.44 v48.88,72.75
DIG3  (via drill 0.35, 0.35 pad 0.55)
  Top 0.305: v8.03,32.86 8,32.89 SEG3.8 8,39.12 v8.26,39.37 | v8,20.5 SEG3.3 | v8.26,66.99 v50.48,66.99 | v50.8,85.72 IC4.7
  Bottom 0.305: v8.03,32.86 8,32.83 v8,20.5 | v50.48,66.99 v50.49,67 50.49,85.41 v50.8,85.72 | v8.26,39.37 v8.26,66.99
DIG4  (via drill 0.35, 0.35 pad 0.55)
  Top 0.305: v22.08,35.24 v22.08,35.25 22.08,37.17 SEG4.8 22,39.15 v22.23,39.37 | v22,20.5 SEG4.3 | v22.23,60.64 v45.95,60.64 | v46.35,90.81 IC4.3
  Bottom 0.305: v22.08,35.24 22.08,20.58 v22,20.5 | v22.23,39.37 v22.23,60.64 | v45.95,60.64 45.98,60.67 45.98,90.43 v46.35,90.81
DIG5  (via drill 0.35, 0.35 pad 0.55)
  Top 0.305: SEG6.8 | SEG6.8 56.67,36.92 | v57,20.5 SEG6.3 | v56.99,39.37 SEG6.8 | v43.18,35.24 43.18,37.07 SEG5.8 43,39.35 v43.02,39.37 | v43,20.5 SEG5.3 | v43.5,48.9 v47.78,48.9 v54.45,48.9 | 53.02,82 IC4.10 v47.78,81.92
  Bottom 0.305: v54.45,48.9 54.45,47.78 56.2,46.04 56.2,40.16 v56.99,39.37 v57,39.36 v57,20.5 | v43.18,35.24 43.18,20.68 v43,20.5 | v43.5,48.9 43.5,39.85 v43.02,39.37 | v47.78,81.92 v47.78,48.9
DIG6  (via drill 0.35, 0.35 pad 0.55)
  Top 0.305: v78,35.25 SEG7.8 78,39.32 v77.95,39.37 | v78,20.5 SEG7.3 | IC4.5 53.12,88.25 v55.25,88.25 | v56.25,77.88 v77.88,77.88
  Bottom 0.305: v78,35.25 v78,20.5 | v77.95,39.37 77.95,77.88 v77.88,77.88 | v56.25,77.88 55.25,78.88 v55.25,88.25
DIG7  (via drill 0.35)
  Top 0.305: v91.92,39.37 92,39.29 SEG8.8 SEG8.3 | v82.07,60.33 v91.92,60.33 | v56.07,84.45 IC4.8 | v56.34,78.73 56.61,78.46 78.12,78.46 78.83,77.75 v82,77.75
  Bottom 0.305: v91.92,60.33 v91.92,39.37 | v56.07,84.45 56.07,79 v56.34,78.73 | v82,77.75 82,60.4 v82.07,60.33
GND  (via drill 0.25, 0.35)
  Top 0.203: IC6.3 31.77,88.33 31.77,88.52 30.91,89.37 | 30.91,89.37 30.56,89.37 IC6.5 | 30.91,89.37 30.75,89.54 v30.75,90.1 | Q4.P$2 36.37,89.64
  Top 0.406: 1.43,81.9 USB1.SHIELD4 0.51,80.97 | USB1.SHIELD2 7.02,80.97 | USB1.SHIELD2 5.61,80.25 | USB1.SHIELD2 4.13,80.97 | USB1.SHIELD3 2.48,89.61 | USB1.SHIELD3 | USB1.SHIELD3 1.43,88.78 | USB1.SHIELD3 0.4,89.61 | USB1.B1/A12 7.22,81.34 | USB1.A1/B12 7.35,89.36 | 7.35,89.36 7.38,89.39 | USB1.SHIELD1 5.61,90.31 | USB1.SHIELD1 7.11,89.61 7.35,89.36 | USB1.SHIELD1 4.25,89.61
  Bottom 0.406: USB1.SHIELD6 1.43,88.82 | USB1.SHIELD6 0.66,89.6 | USB1.SHIELD6 2.58,89.6 | USB1.SHIELD5 4.48,89.6 | USB1.SHIELD5 7,89.6 | USB1.SHIELD5 5.62,88.82 | USB1.SHIELD5 | 5.61,90.47 USB1.SHIELD5 | USB1.SHIELD2 5.61,80.21 | USB1.SHIELD2 6.71,80.97 | USB1.SHIELD2 4.08,80.97 | USB1.SHIELD4 1.43,81.86 | USB1.SHIELD4 2.57,80.97 | USB1.SHIELD4 0.56,80.97
  other vias: 14.84,80.96 16.31,84.38 21.31,86.44 24.41,80.8 33.54,86.64 27.89,91.33 10.48,85.01 4.48,79.89 3.37,87.35 3.33,85.29 41,90.37 30.72,79.38 35.6,92.15 35.04,81.99 27.02,88.71 7.41,89.43 8.24,86.85 13.05,86.77 15.17,86.67 3.84,81.93 1.42,87.25 1.34,83.32 45,13 53,35.5 10.5,4 45.5,3 80.5,3 26.67,96.04 65.74,58.74 46.75,77 70.75,91.44 70.75,90.19 70.75,88.94 70.69,83.81 70.69,82.56 70.69,81.25 28.12,0.62 50.81,92.75 50.81,91.44 51.12,81.31 51.12,80 64.56,80 64.56,81.31 64.56,82.56 64.56,83.81 64.88,88.88 64.88,90.19 64.88,91.44 41.5,49
  pour Top: -0.5,100.5 -0.5,-0.5 100.5,-0.5 100.5,100.5
  pour Bottom: 100.5,100.5 100.5,-0.5 -0.5,-0.5 -0.5,100.5
N$1
  Top 0.203: C8.1 12.19,81.84 11.87,82.15 IC5.4
N$2
  Top 0.203: C9.1 18.34,86.58 18.23,86.58 | 18.23,86.58 Q3.P$1 | IC5.7 15.68,86.17 16.1,86.58 18.23,86.58
N$3
  Top 0.203: C10.1 20.1,84.31 Q3.P$3 20.07,85.34 19.92,85.49 17.46,85.49 16.95,84.98 IC5.8
N$4
  Top 0.203: C15.2 15.32,81.24 15.08,81.47 15.08,84.45 14.61,84.93 12.22,84.93 11.87,85.28 IC5.13
N$5  (via drill 0.25)
  Top 0.203: IC5.5 13.14,84.01 12.88,84.27 9.66,84.27 v9.6,84.22 | R8.2 9.91,81.29 v9.6,81.6
  Bottom 0.203: v9.6,81.6 v9.6,84.22
N$6  (via drill 0.35)
  Top 0.61: R2.1 v57.47,76.75 | v57.47,85.72 IC4.18
  Bottom 0.61: v57.47,76.75 v57.47,85.72
N$7  (via drill 0.35)  (1 unrouted)
  Top 0.61: 73.66,84.23 R1.2 v73.66,79.38 | 73.73,84.3 74.66,85.23 R1.1 | v73.66,76.83 73.58,76.75 R2.2
  Bottom 0.61: v73.66,79.38 v73.66,76.83
N$8
  Top 0.203: IC5.6 14.41,84.25 14.06,84.6 11.75,84.6 11.25,85.1 11.25,89.79 R9.2
N$9  (via drill 0.45)
  Top 0.406: USB1.A4/B9 5.75,87.74 5.28,87.27 v4.63,87.27 3.49,88.42 3.49,90.49 2.82,91.16 L2.1 | USB1.B4/A9 5.75,82.84 5.32,83.27 v4.55,83.27
  Bottom 0.406: v4.55,83.27 4.55,87.19 v4.63,87.27
N$10
  Top 0.203: USB1.B5 5.74,83.54 4.95,84.33 3.21,84.33 2.87,83.99 2.87,80.02 2.24,79.39 R10.2
N$11
  Top 0.203: USB1.A5 3.11,86.54 2.54,85.97 2.54,80.25 2.3,80.01 1.27,80.01 0.87,79.61 R11.2
N$12
  Top 0.203: C24.1 34.56,87.19 Q4.P$1 34.14,88.69 34.14,89.21 32.56,90.79 30.58,90.79 30.43,90.64 29.56,90.64 IC6.7
N$13
  Top 0.203: IC6.8 28.83,91.04 30.29,91.04 30.37,91.13 32.71,91.13 33.02,91.44 33.37,91.44 33.84,90.97 33.84,90.89 Q4.P$3 34.49,91.44 34.92,91.44 35.91,90.46 C25.1
RESET  (via drill 0.25, 0.3)
  Top 0.203: v25.82,83.35 v25.83,83.34 30.1,83.34 IC6.29 31.51,81.93 31.51,80.29 | C15.1 18.41,81.24 18.79,81.61 v18.79,81.85 | 31.51,80.29 31.51,79.69 32.05,79.16 34.29,79.16 | R12.2 31.52,80.3 31.51,80.29 | 38.46,79.16 34.29,79.16 | ISP1.5 38.13,81.57 38.46,81.24 38.46,79.16 | U$2.RST 34.3,79.15 34.29,79.16 | U$2.RST1 34.97,92.91 35.12,92.76 35.12,91.95 35.88,91.19 41.69,91.19 42.03,90.84 42.03,79.33 41.85,79.16 38.46,79.16
  Bottom 0.203: v18.79,81.85 24.32,81.85 v25.82,83.35
SEG1  (via drill 0.35, 0.35 pad 0.55)  (1 unrouted)
  Top 0.305: 80.49,41.27 v93.34,41.27 94.46,41.27 94.54,41.19 SEG8.7 94.76,37.47 | 10.65,37.36 SEG3.7 10.54,41.16 10.65,41.27 v24.62,41.27 v40.02,41.27 v45.72,41.27 v59.69,41.27 59.85,41.43 v64.72,41.43 80.33,41.43 80.49,41.27 | v24.62,39.37 24.62,37.33 SEG4.7 | v45.72,39.37 45.56,39.21 45.56,37.27 SEG5.7 | 59.69,37.4 SEG6.7 59.54,39.22 v59.69,39.37 | 80.79,37.5 SEG7.7 80.54,41.22 80.49,41.27 | v63.57,68.42 63.54,68.45 SEG2.7 | SEG1.7 41.54,68.45 v41.51,68.42 | IC4.14 v67.94,80.64
  Bottom 0.305: v24.62,41.27 v24.62,39.37 | v45.72,41.27 v45.72,39.37 | v59.69,39.37 v59.69,41.27 | v67.94,80.64 92.71,80.64 93.34,80.01 v93.34,41.27 | v63.57,68.42 63.57,59.22 64.72,58.08 v64.72,41.43 | v41.51,68.42 41.51,59.42 40.02,57.94 v40.02,41.27
SEG2  (via drill 0.35, 0.35 pad 0.55)  (1 unrouted)
  Top 0.305: v13.19,42.23 v27.16,42.23 27.18,42.25 v42.62,42.25 48.24,42.25 v48.26,42.23 v61.73,42.23 v67.43,42.23 v83.03,42.23 v94.61,42.23 96.86,42.23 97.08,42.01 SEG8.6 97.3,37.47 | SEG3.6 13.1,37.27 13.1,39.29 v13.18,39.37 | SEG4.6 27.16,37.33 v27.16,39.37 | SEG5.6 48.26,37.43 v48.26,39.37 | 62.23,37.4 SEG6.6 62.08,39.02 v61.73,39.37 | 83.33,37.5 SEG7.6 83.08,39.32 v83.03,39.37 | v66.11,68.42 66.08,68.45 SEG2.6 | SEG1.6 44.08,68.45 v44.05,68.42 | IC4.16 v67.94,83.19
  Bottom 0.305: v13.19,42.23 13.18,42.21 v13.18,39.37 | v27.16,39.37 v27.16,42.23 | v48.26,39.37 v48.26,42.23 | v61.73,42.23 v61.73,39.37 | v83.03,42.23 v83.03,39.37 | v66.11,68.42 66.11,59.5 67.46,58.15 67.46,43.04 67.43,43.02 v67.43,42.23 | v44.05,68.42 44.05,59.42 42.69,58.06 42.69,42.31 v42.62,42.25 | v67.94,83.19 93.71,83.19 94.61,82.28 v94.61,42.23
SEG3  (via drill 0.35, 0.35 pad 0.55)  (1 unrouted)
  Top 0.305: v9.06,43.18 v23.04,43.18 23.16,43.05 v42.07,43.05 44.01,43.05 v44.13,43.18 v58.1,43.18 v64.06,43.18 v79.2,43.18 v93.98,43.18 v95.89,43.18 | SEG3.4 10.54,20.46 v10.5,20.5 | SEG4.4 24.5,18.79 v24.5,20.5 | SEG5.4 45.5,18.79 v45.5,20.5 | SEG6.4 59.5,18.79 v59.5,20.5 | SEG7.4 80.54,20.46 v80.5,20.5 | SEG8.4 94.54,20.46 v94.5,20.5 | v63.64,50.01 63.54,50.1 SEG2.4 | SEG1.4 41.54,50.04 v41.5,50 | v67.94,88.27 IC4.20
  Bottom 0.305: v10.5,20.5 10.5,26 9.06,27.43 v9.06,43.18 | v24.5,20.5 24.5,26.58 23.04,28.04 v23.04,43.18 | v45.5,20.5 45.5,26.5 44.13,27.87 v44.13,43.18 | v59.5,20.5 59.5,26.25 58.1,27.65 v58.1,43.18 | v80.5,20.5 80.5,27 79.2,28.3 v79.2,43.18 | v94.5,20.5 93.98,21.02 v93.98,43.18 | v42.07,43.05 42.19,43.18 42.19,49.31 v41.5,50 | v95.89,43.18 95.89,86.09 93.71,88.27 v67.94,88.27 | v64.06,43.18 64.06,49.59 v63.64,50.01
SEG4  (via drill 0.35, 0.35 pad 0.55)
  Top 0.305: v6.84,44.13 v17.95,44.13 v36.87,44.13 v41.59,44.13 v55.56,44.13 v55.57,44.12 v58.5,44.12 v76.65,44.12 v76.66,44.13 v90.63,44.13 v97.79,44.13 | SEG3.2 5.46,20.29 v5.25,20.5 | SEG4.2 19.46,20.46 v19.5,20.5 | SEG5.2 40.46,20.46 v40.5,20.5 | SEG6.2 54.46,20.46 v54.5,20.5 | SEG7.2 75.46,20.29 v75.25,20.5 | SEG8.2 89.46,20.46 v89.5,20.5 | SEG2.2 58.46,50.04 v58.49,50.01 | SEG1.2 36.46,50.04 v36.43,50.01 | v67.94,92.08 IC4.23
  Bottom 0.305: v6.84,44.13 6.84,27.34 5.25,25.75 v5.25,20.5 | v19.5,20.5 19.5,26.09 17.95,27.63 v17.95,44.13 | v40.5,20.5 40.5,26.5 41.47,27.47 41.47,44.01 v41.59,44.13 | v55.56,44.13 55.56,27.31 54.5,26.25 v54.5,20.5 | v75.25,20.5 75.25,26.75 76.66,28.16 v76.66,44.13 | v90.63,44.13 90.63,28.13 89.5,27 v89.5,20.5 | v67.94,92.08 93.71,92.08 97.79,88 v97.79,44.13 | v58.49,50.01 58.52,49.97 58.52,44.15 v58.5,44.12 | v36.43,50.01 36.87,49.56 v36.87,44.13
SEG5  (via drill 0.35, 0.35 pad 0.55)
  Top 0.305: v1.75,45.09 v14.46,45.09 v33.35,45.09 v36.2,45.09 v51.12,45.09 v57.31,45.09 v71.26,45.09 v87.93,45.09 88.02,45 v96.5,45 | v2.75,20.5 2.92,20.33 SEG3.1 | SEG4.1 16.92,20.33 v16.75,20.5 | SEG5.1 37.92,20.33 v37.75,20.5 | SEG6.1 51.92,20.33 v51.75,20.5 | SEG7.1 72.92,20.33 v72.75,20.5 | SEG8.1 86.92,20.33 v86.75,20.5 | v56.02,50.01 55.92,50.1 SEG2.1 | v67.94,89.53 IC4.21 | v33.75,50 33.75,50.03 33.92,50.2 SEG1.1
  Bottom 0.305: v2.75,20.5 2.75,26.25 1.76,27.24 1.76,45.07 v1.75,45.09 | v16.75,20.5 16.75,33.91 14.46,36.2 v14.46,45.09 | v37.75,20.5 37.75,26.5 36.2,28.05 v36.2,45.09 | v51.75,20.5 51.75,26.5 51.12,27.13 v51.12,45.09 | v72.75,20.5 72.75,26.25 71.26,27.74 v71.26,45.09 | v87.93,45.09 87.93,28.08 86.75,26.9 v86.75,20.5 | v56.02,50.01 56.02,47.49 57.31,46.2 v57.31,45.09 | v33.75,50 33.75,45.48 v33.35,45.09 | v96.5,45 96.5,86.75 93.71,89.53 v67.94,89.53
SEG6  (via drill 0.35, 0.35 pad 0.55)  (1 unrouted)
  Top 0.305: v5.89,46.04 v18.91,46.04 v35.38,46.04 v40.64,46.04 v54.61,46.04 54.77,46.2 v59.71,46.2 75.55,46.2 v75.71,46.04 v89.68,46.04 v93.98,46.04 | 5.57,37.36 SEG3.9 5.46,39.26 v5.57,39.37 | SEG4.9 19.46,39.32 v19.32,39.46 | SEG5.9 40.64,37.43 v40.64,39.37 | SEG6.9 54.61,37.4 v54.61,39.37 | SEG7.9 75.71,37.5 v75.71,39.37 | 89.68,37.47 SEG8.9 89.46,39.3 v89.53,39.37 | SEG2.9 58.46,68.45 v58.49,68.42 | SEG1.9 36.46,68.45 v36.43,68.42 | v67.94,81.92 IC4.15
  Bottom 0.305: v5.89,46.04 5.89,39.69 v5.57,39.37 | v19.32,39.46 18.91,39.87 v18.91,46.04 | v40.64,39.37 v40.64,46.04 | v54.61,39.37 v54.61,46.04 | v75.71,39.37 v75.71,46.04 | v89.68,46.04 89.53,45.9 v89.53,39.37 | v58.49,68.42 58.49,59.21 59.71,58 v59.71,46.2 | v36.43,68.42 36.43,59.42 35.38,58.38 v35.38,46.04 | v93.98,46.04 93.98,80.96 93.03,81.92 v67.94,81.92
SEG7  (via drill 0.35, 0.35 pad 0.55)  (1 unrouted)
  Top 0.305: v3.19,46.99 v17,46.99 v34.43,46.99 v38.73,46.99 v52.07,46.99 v57.67,46.99 v73.17,46.99 v87.14,46.99 v95.25,46.99 | 3.12,37.45 SEG3.10 2.92,39.17 v3.12,39.37 | SEG4.10 17,37.33 v17,39.37 | SEG5.10 38.1,37.43 v38.1,39.37 | SEG6.10 52.07,37.4 v52.07,39.37 | SEG7.10 73.17,37.5 v73.17,39.37 | 87.14,37.47 SEG8.10 86.92,39.3 v87,39.37 | SEG2.10 55.92,68.45 v55.95,68.42 | SEG1.10 33.92,68.55 v34.05,68.42 | v67.94,84.45 IC4.17
  Bottom 0.305: v3.12,39.37 3.19,39.44 v3.19,46.99 | v17,39.37 v17,46.99 | v38.73,46.99 38.73,40.01 v38.1,39.37 | v52.07,39.37 v52.07,46.99 | v73.17,39.37 v73.17,46.99 | v87,39.37 87,46.85 v87.14,46.99 | v55.95,68.42 55.95,59.21 57.42,57.75 57.42,47.24 v57.67,46.99 | v34.05,68.42 34.5,67.97 34.5,47.06 v34.43,46.99 | v95.25,46.99 95.25,82.92 93.71,84.45 v67.94,84.45
SEG8  (via drill 0.35, 0.35 pad 0.55)
  Top 0.305: v11.92,47.94 12.08,47.78 v27.8,47.78 27.83,47.82 v44.37,47.82 46.87,47.82 v46.99,47.94 v62.46,47.94 v66,47.94 v83.66,47.94 v97.16,47.94 | SEG3.5 13.08,20.42 v13,20.5 | SEG5.5 48.08,20.42 v48,20.5 | SEG4.5 27.08,20.42 v27,20.5 | SEG6.5 62.08,20.42 v62,20.5 | SEG7.5 83.08,20.42 v83,20.5 | SEG8.5 97.08,20.42 v97,20.5 | 66.38,51.75 SEG2.5 66.08,50.08 v66,50 | v44.12,50.01 44.08,50.04 SEG1.5 | IC4.22 v67.94,90.81
  Bottom 0.305: v13,20.5 13,26 12,27 12,47.87 v11.92,47.94 | v48,20.5 48,26.5 47,27.5 47,46.68 46.99,46.69 v46.99,47.94 | v27.8,47.78 v27.79,47.78 27.79,27.33 27,26.53 v27,20.5 | v62.46,47.94 62.46,26.69 62,26.23 v62,20.5 | v83.66,47.94 83.66,21.16 v83,20.5 | v97,20.5 97.16,20.66 v97.16,47.94 97.16,87.36 93.71,90.81 v67.94,90.81 | v44.12,50.01 44.37,49.76 v44.37,47.82 | v66,50 v66,47.94

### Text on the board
Bottom: multiplication-trainer_1.0 RevA
tPlace: D12 | D11 | D10 | D9 | D8 | D7 | D6 | D5 | D4 | D3 | D2 | GND | RST | D0 | D1 | BRIGHTNESS | JLCJLCJLCJLC | D13 | +3V3 | AREF | A0 | A1 | A2 | A3 | A4 | A5 | A6 | A7 | +5V | RST | GND | VIN | =?
bStop: multiplication-trainer_1.0 RevA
